[IBIS Ver]   3.2
[File Name]   sprm297.ibs
[File Rev]   1.0
[Date]   November 3, 2003
[Source]   File originated at Texas Instruments
[Copyright]   (c) 2003, Texas Instruments Inc.
[Component]   f2812ghh
[Manufacturer] Texas Instruments
[Package]
| Variable   Typ   Min   Max
R_pkg   0.08821   0.00445   0.1444
L_pkg   2.312e-09   3.373e-10   3.933e-09
C_pkg   2.855e-13   1.279e-13   4.259e-13
[Pin] signal_name   model_name   R_pin   L_pin   C_pin
B2   VDDAIO   NC   0.09209  2.36e-09   2.324e-13
C2   ADCINB0   ioh125   0.08702  2.145e-09  2.491e-13
C3   ADCINB1   ioh125   0.08455  2.129e-09  2.412e-13
B1   ADCINB2   ioh125   0.1237   3.291e-09  3.802e-13
C1   ADCINB3   ioh125   0.103   2.673e-09  3.339e-13
D3   ADCINB4   ioh125   0.07884  2.005e-09  2.389e-13
D2   ADCINB5   ioh125   0.07849  1.946e-09  2.548e-13
D1   ADCINB6   ioh125   0.09972  2.597e-09  2.918e-13
F5   ADCINB7   ioh125   0.1392   3.811e-09  4.225e-13
E4   ADCREFM   ioh125   0.1002   2.62e-09   3.512e-13
E2   ADCREFP   ioh125   0.07253  1.807e-09  2.304e-13
E3   AVSSREFBG   ioh125   0.07152  1.838e-09  2.399e-13
E1   AVDDREFBG   ioh125   0.09207  2.431e-09  2.756e-13
F4   VDDA1   NC   0.09478  2.501e-09  3.059e-13
F3   VSSA1   NC   0.06871  1.775e-09  2.4e-13
F2   ADCRESEXT   ioh125   0.06839  1.711e-09  2.218e-13
F1   XMPNMC   idg095_pe1005   0.09079  2.383e-09  2.69e-13
G5   XA(0)   oui835   0.1124   3.004e-09  3.787e-13
G4   VSS   NC   0.09241  2.449e-09  3.276e-13
G2   MDRA   idg095_ouo435_ps1005  0.06703  1.677e-09  2.109e-13
G3   XD(0)   idg095_oui835_ps1005  0.06663  1.72e-09   2.244e-13
G1   MDXA   idg095_ouo435   0.08649  2.3e-09   3.064e-13
H1   VDD   NC   0.08687  2.308e-09  3.051e-13
H3   XD(1)   idg095_oui835_ps1005  0.0675   1.739e-09  2.278e-13
H2   MCLKRA   idg095_ouo435_ps1005  0.06857  1.71e-09   2.172e-13
H4   MFSXA   idg095_ouo435_ps1005  0.0958   2.514e-09  3.319e-13
H5   XD(2)   idg095_oui835_ps1005  0.1148   3.076e-09  3.819e-13
J1   MCLKXA   idg095_ouo435_ps1005  0.09444  2.462e-09  2.835e-13
J2   MFSRA   idg095_ouo435_ps1005  0.07272  1.804e-09  2.338e-13
J3   XD(3)   idg095_oui835_ps1005  0.07371  1.889e-09  2.436e-13
J4   VDDIO   NC   0.09822  2.576e-09  3.054e-13
K1   VSS   NC   0.09654  2.518e-09  2.844e-13
K3   XD(4)   idg095_oui835_ps1005  0.07688  1.955e-09  2.515e-13
K2   SPICLKA   idg095_ouo435   0.07656  1.898e-09  2.333e-13
K4   SPISTEA   idg095_ouo435   0.1045   2.711e-09  3.594e-13
J5   XD(5)   idg095_oui835_ps1005  0.1444   3.933e-09  4.259e-13
L1   VDD   NC   0.1023   2.666e-09  2.93e-13
L2   VSS   NC   0.08196  2.025e-09  2.536e-13
L3   XD(6)   idg095_oui835_ps1005  0.08003  2.035e-09  2.292e-13
M1   SPISIMOA   idg095_ouo435   0.1022   2.66e-09   3.169e-13
N1   SPISOMIA   idg095_ouo435   0.1206   3.247e-09  3.719e-13
M3   XRDn   oui835   0.08199  2.072e-09  2.38e-13
M2   XA(1)   oui835   0.08514  2.104e-09  2.563e-13
P1   XZCS0AND1n   oui835   0.1272   3.432e-09  3.17e-13
N2   PWM7   sw0145_ouo435_ups285  0.09249  2.375e-09  2.344e-13
P2   PWM8   sw0145_ouo435_ups285  0.1091   2.835e-09  3.24e-13
N3   PWM9   sw0145_ouo435_ups285  0.0847   2.1e-09   2.977e-13
P3   PWM10   sw0145_ouo435_ups285  0.1058   2.786e-09  3.224e-13
L4   PWM11   sw0145_ouo435_ups285  0.1017   2.696e-09  3.056e-13
M4   PWM12   sw0145_ouo435_ups285  0.07819  1.991e-09  2.576e-13
N4   XRNW   oui835   0.07522  1.886e-09  2.531e-13
P4   VSS   NC   0.09848  2.623e-09  3.028e-13
K5   T3PWM_T3CMP   sw0145_ouo435_ups285  0.1128   3.022e-09  3.435e-13
L5   XD(7)   idg095_oui835_ps1005  0.09136  2.382e-09  3.006e-13
N5   T4PWM_T4CMP   sw0145_ouo435_ups285  0.06842  1.716e-09  2.385e-13
P5   VDD   NC   0.09175  2.499e-09  2.855e-13
M5   CAP4_QEP3   sw0145_ouo435_ups285  0.05893  1.5e-09   2.17e-13
K6   VSS   NC   0.1035   2.805e-09  3.409e-13
M6   CAP5_QEP4   sw0145_ouo435_ups285  0.06207  1.604e-09  2.311e-13
P6   CAP6_QEPI2   sw0145_ouo435_ups285  0.09133  2.468e-09  2.967e-13
N6   C4TRIPn   sw0145_ouo435_ups285  0.06341  1.612e-09  2.156e-13
L6   C5TRIPn   sw0145_ouo435_ups285  0.08399  2.26e-09   3.049e-13
K7   C6TRIPn   sw0145_ouo435_ups285  0.1038   2.828e-09  3.985e-13
L7   VDDIO   NC   0.08372  2.239e-09  3.16e-13
P7   XD(8)   idg095_oui835_ps1005  0.0865   2.353e-09  2.75e-13
N7   TEST2   iog195   0.06169  1.56e-09   2.049e-13
M7   TEST1   iog195   0.06268  1.695e-09  2.38e-13
M8   XD(9)   idg095_oui835_ps1005  0.06259  1.694e-09  2.398e-13
N8   VDD3VFL   NC   0.0611   1.546e-09  2.12e-13
P8   VSS   NC   0.08825  2.433e-09  2.701e-13
L8   TDIRB   sw0145_ouo435_ups285  0.08293  2.235e-09  3.129e-13
K8   TCLKINB   sw0145_ouo435_ups285  0.102   2.793e-09  3.815e-13
L9   XD(10)   idg095_oui835_ps1005  0.0859   2.316e-09  3.071e-13
N9   XD(11)   idg095_oui835_ps1005  0.06134  1.562e-09  2.256e-13
P9   VDD   NC   0.08678  2.402e-09  2.814e-13
M9   X2   NC   0.05751  1.488e-09  2.185e-13
K9   X1/XCLKIN   NC   0.1051   2.874e-09  3.416e-13
M10   VSS   NC   0.06466  1.77e-09   2.525e-13
P10   T3CTRIP_PDPINTBn idg095_ouo435_ps1005  0.09255  2.499e-09  2.906e-13
N10   XA(2)   oui835   0.06746  1.702e-09  2.398e-13
L10   VDDIO   NC   0.09217  2.446e-09  3.236e-13
K10   XHOLDAn   oui835   0.1143   3.12e-09   3.69e-13
P11   T4CTRIPn/EVBSOCn idg095_ouo435_ps1005  0.09684  2.574e-09  2.997e-13
N11   XWEn   oui835   0.07403  1.857e-09  2.454e-13
M11   XA(3)   oui835   0.07441  1.903e-09  2.389e-13
L11   VSS   NC   0.104   2.76e-09   3.07e-13
P12   VDD   NC   0.103   2.706e-09  3.157e-13
N12   CANTXA   idg095_ouo435_ps1005  0.08258  2.052e-09  2.669e-13
P13   XZCS2n   oui835   0.1083   2.856e-09  2.829e-13
N13   CANRXA   idg095_ouo435_ps1005  0.09197  2.37e-09   2.499e-13
P14   SCITXDB   idg095_ouo435   0.1255   3.388e-09  3.392e-13
M13   SCIRXDB   idg095_ouo435   0.08237  2.039e-09  2.548e-13
M12   PWM1   idg095_ouo435_ps1005  0.08225  2.075e-09  2.456e-13
N14   VDDIO   NC   0.1201   3.231e-09  3.81e-13
M14   PWM2   idg095_ouo435_ps1005  0.09891  2.59e-09   3.294e-13
L12   PWM3   idg095_ouo435_ps1005  0.07898  2.006e-09  2.447e-13
L13   PWM4   idg095_ouo435_ps1005  0.07487  1.867e-09  2.444e-13
L14   XD(12)   idg095_oui835_ps1005  0.09893  2.587e-09  2.886e-13
J10   XD(13)   idg095_oui835_ps1005  0.1386   3.798e-09  4.176e-13
K11   PWM5   idg095_ouo435_ps1005  0.09954  2.607e-09  3.482e-13
K13   VSS   NC   0.0709   1.771e-09  2.325e-13
K12   VDD   NC   0.07034  1.811e-09  2.401e-13
K14   PWM6   idg095_ouo435_ps1005  0.09406  2.475e-09  2.775e-13
J11   T1PWM_T1CMP   idg095_ouo435_ps1005  0.09311  2.447e-09  3.027e-13
J12   XA(4)   oui835   0.0707   1.815e-09  2.418e-13
J13   T2PWM_T2CMP   idg095_ouo435_ps1005  0.06707  1.681e-09  2.219e-13
J14   VSS   NC   0.09108  2.388e-09  2.791e-13
H10   CAP1_QEP1   idg095_ouo435_ps1005  0.1139   3.036e-09  3.844e-13
H11   CAP2_QEP2   idg095_ouo435_ps1005  0.09328  2.466e-09  3.308e-13
H13   XA(5)   oui835   0.06503  1.629e-09  2.144e-13
H12   CAP3_QEPI1   idg095_ouo435_ps1005  0.06577  1.702e-09  2.25e-13
H14   T1CTRIP_PDPINTAn idg095_ouo435_ps1005  0.08639  2.297e-09  3.03e-13
G14   XA(6)   oui835   0.0873   2.319e-09  3.041e-13
G12   VDD   NC   0.06918  1.777e-09  2.274e-13
G13   VSS   NC   0.06778  1.692e-09  2.146e-13
G11   VDDIO   NC   0.09314  2.459e-09  3.346e-13
G10   T2CTRIPn/EVASOCn idg095_ouo435_ps1005  0.1138   3.052e-09  3.802e-13
F14   TDIRA   idg095_ouo435_ps1005  0.09404  2.462e-09  2.798e-13
F13   TCLKINA   idg095_ouo435_ps1005  0.06786  1.696e-09  2.218e-13
F12   XA(7)   oui835   0.07232  1.856e-09  2.474e-13
F11   XCLKOUT   oui835   0.09426  2.507e-09  3.058e-13
E14   VSS   NC   0.09525  2.497e-09  2.91e-13
E12   XA(8)   oui835   0.07626  1.938e-09  2.582e-13
E13   C1TRIPn   idg095_ouo435_ps1005  0.07579  1.878e-09  2.366e-13
E11   C2TRIPn   idg095_ouo435_ps1005  0.1028   2.672e-09  3.561e-13
F10   C3TRIPn   idg095_ouo435_ps1005  0.1414   3.864e-09  4.252e-13
D14   XA(9)   oui835   0.1035   2.69e-09   2.981e-13
D13   TMS   idg095_ps1005   0.07795  1.936e-09  2.479e-13
D12   TDO   oui835   0.08151  2.062e-09  2.503e-13
C14   VDD   NC   0.1046   2.725e-09  3.442e-13
B14   VSS   NC   0.1242   3.313e-09  3.855e-13
C12   XA(10)   oui835   0.08905  2.226e-09  2.563e-13
C13   TDI   idg095_ps1005   0.0903   2.216e-09  2.631e-13
A14   XA(11)   oui835   0.1281   3.455e-09  3.132e-13
B13   XZCS6AND7n   oui835   0.09387  2.397e-09  2.377e-13
A13   TESTSEL   idg095_pe1005   0.1042   2.726e-09  3.249e-13
B12   TRSTn   idg095_pe1005   0.00445  3.373e-10  1.279e-13
A12   TCK   idg095_ps1005   0.1012   2.679e-09  3.184e-13
D11   EMU0   idg095_oui835_ps1005  0.09979  2.649e-09  3.147e-13
C11   XA(12)   oui835   0.07303  1.881e-09  2.526e-13
B11   XD(14)   idg095_oui835_ps1005  0.07161  1.807e-09  2.388e-13
A11   XF_XPLLDIS   idg095_oui835_ps1005  0.09603  2.567e-09  2.922e-13
E10   XA(13)   oui835   0.1156   3.087e-09  3.455e-13
D10   VSS   NC   0.09186  2.405e-09  2.985e-13
B10   VDD   NC   0.06885  1.731e-09  2.29e-13
A10   XA(14)   oui835   0.09485  2.561e-09  2.856e-13
C10   VSS   NC   0.063988 1.613e-09  2.243e-13
E9   VDDIO   NC   0.1082   2.906e-09  3.452e-13
C9   EMU1   idg095_oui835_ps1005  0.06274  1.614e-09  2.346e-13
A9   XD(15)   idg095_oui835_ps1005  0.09338  2.506e-09  3.182e-13
B9   XA(15)   oui835   0.06408  1.62e-09   2.367e-13
D9   XINT1_XBIOn   idg095_ouo435   0.08668  2.311e-09  3.397e-13
E8   XNMI_XINT13   idg095_ouo435_ps1005  0.1043   2.833e-09  3.974e-13
D8   XINT2_ADCSOC   idg095_ouo435   0.08381  2.248e-09  3.111e-13
A8   XA(16)   oui835   0.08698  2.367e-09  2.747e-13
B8   VSS   NC   0.06146  1.548e-09  2.203e-13
C8   VDD   NC   0.0627   1.691e-09  2.545e-13
C7   SCITXDA   idg095_ouo435_ps1005  0.06257  1.689e-09  2.491e-13
B7   XA(17)   oui835   0.06157  1.552e-09  2.151e-13
A7   SCIRXDA   idg095_ouo435_ps1005  0.08827  2.43e-09   2.835e-13
D7   XA(18)   oui835   0.08506  2.269e-09  3.34e-13
E7   XHOLDn   idg095_ps1005   0.1043   2.826e-09  3.994e-13
D6   XRSn   idg095_oum425_ps1005  0.08576  2.305e-09  3.177e-13
B6   XREADY   idg095_ps1005   0.0641   1.621e-09  2.324e-13
A6   VDD1   NC   0.09005  2.472e-09  2.845e-13
C6   VSS1   NC   0.06117  1.569e-09  2.29e-13
E6   ADCBGREFIN   ioh125   0.1067   2.898e-09  3.505e-13
C5   VSSA2   NC   0.06463  1.768e-09  2.521e-13
A5   VDDA2   NC   0.09355  2.521e-09  2.935e-13
B5   ADCINA7   ioh125   0.06979  1.749e-09  2.589e-13
D5   ADCINA6   ioh125   0.09531  2.493e-09  3.268e-13
E5   ADCINA5   ioh125   0.115   3.131e-09  3.515e-13
A4   ADCINA4   ioh125   0.101   2.662e-09  3.031e-13
B4   ADCINA3   ioh125   0.07696  1.923e-09  2.515e-13
C4   ADCINA2   ioh125   0.0785   1.993e-09  2.483e-13
D4   ADCINA1   ioh125   0.1037   2.755e-09  3.086e-13
A3   ADCINA0   ioh125   0.1053   2.763e-09  3.109e-13
B3   ADCLO   ioh125   0.08665  2.149e-09  2.561e-13
A2   VSSAIO   NC   0.1087   2.841e-09  2.701e-13
| End of package information
| Component idg095
[Component]   idg095
[Manufacturer]   Texas Instruments
[Package]
|   typ   min   max
R_pkg   0   0   0
L_pkg   0   0   0
C_pkg   0   0   0
[Pin]   signal_name   model_name   R_pin   L_pin   C_pin
   1   A   idg095   0   0   0
| Component idg095_oui835_ps1005
[Component]   idg095_oui835_ps1005
[Manufacturer]   Texas Instruments
[Package]
|   typ   min   max
R_pkg   0   0   0
L_pkg   0   0   0
C_pkg   0   0   0
[Pin]   signal_name   model_name   R_pin   L_pin   C_pin
   1   Y  idg095_oui835_ps1005   0   0   0
| Component idg095_oum425_ps1005
[Component]   idg095_oum425_ps1005
[Manufacturer]   Texas Instruments
[Package]
|   typ   min   max
R_pkg   0   0   0
L_pkg   0   0   0
C_pkg   0   0   0
[Pin]   signal_name   model_name   R_pin   L_pin   C_pin
   1   Y  idg095_oum425_ps1005   0   0   0
| Component idg095_ouo435_ps1005
[Component]   idg095_ouo435_ps1005
[Manufacturer]   Texas Instruments
[Package]
|   typ   min   max
R_pkg   0   0   0
L_pkg   0   0   0
C_pkg   0   0   0
[Pin]   signal_name   model_name   R_pin   L_pin   C_pin
   1   Y  idg095_ouo435_ps1005   0   0   0
| Component idg095_pe1005
[Component]   idg095_pe1005
[Manufacturer]   Texas Instruments
[Package]
|   typ   min   max
R_pkg   0   0   0
L_pkg   0   0   0
C_pkg   0   0   0
[Pin]   signal_name   model_name   R_pin   L_pin   C_pin
   1   A   idg095_pe1005   0   0   0
| Component idg095_ps1005
[Component]   idg095_ps1005
[Manufacturer]   Texas Instruments
[Package]
|   typ   min   max
R_pkg   0   0   0
L_pkg   0   0   0
C_pkg   0   0   0
[Pin]   signal_name   model_name   R_pin   L_pin   C_pin
   1   A   idg095_ps1005   0   0   0
| Component iog195
[Component]   iog195
[Manufacturer]   Texas Instruments
[Package]
|   typ   min   max
R_pkg   0   0   0
L_pkg   0   0   0
C_pkg   0   0   0
[Pin]   signal_name   model_name   R_pin   L_pin   C_pin
   1   Y   iog195   0   0   0
| Component ioh125
[Component]   ioh125
[Manufacturer]   Texas Instruments
[Package]
|   typ   min   max
R_pkg   0   0   0
L_pkg   0   0   0
C_pkg   0   0   0
[Pin]   signal_name   model_name   R_pin   L_pin   C_pin
   1   Y   ioh125   0   0   0
| Component oui835
[Component]   oui835
[Manufacturer]   Texas Instruments
[Package]
|   typ   min   max
R_pkg   0   0   0
L_pkg   0   0   0
C_pkg   0   0   0
[Pin]   signal_name   model_name   R_pin   L_pin   C_pin
   1   Y   oui835   0   0   0
| Component oum425
[Component]   oum425
[Manufacturer]   Texas Instruments
[Package]
|   typ   min   max
R_pkg   0   0   0
L_pkg   0   0   0
C_pkg   0   0   0
[Pin]   signal_name   model_name   R_pin   L_pin   C_pin
   1   Y   oum425   0   0   0
| Component idg095_ouo435
[Component]   idg095_ouo435
[Manufacturer]   Texas Instruments
[Package]
|   typ   min   max
R_pkg   0   0   0
L_pkg   0   0   0
C_pkg   0   0   0
[Pin]   signal_name   model_name   R_pin   L_pin   C_pin
   1   Y   idg095_ouo435   0   0   0
| Component ouo435
[Component]   ouo435
[Manufacturer]   Texas Instruments
[Package]
|   typ   min   max
R_pkg   0   0   0
L_pkg   0   0   0
C_pkg   0   0   0
[Pin]   signal_name   model_name   R_pin   L_pin   C_pin
   1   Y   ouo435   0   0   0
| Component sw0145_ouo435_ups285
[Component]   sw0145_ouo435_ups285
[Manufacturer]   Texas Instruments
[Package]
|   typ   min   max
R_pkg   0   0   0
L_pkg   0   0   0
C_pkg   0   0   0
[Pin]   signal_name   model_name   R_pin   L_pin   C_pin
   1   Y  sw0145_ouo435_ups285   0   0   0
| Models and submodels in the file (13): idg095 (Input), idg095_oui835_ps1005 (I/O), idg095_oum425_ps1005 (I/O_open_sink), idg095_ouo435_ps1005 (I/O), idg095_pe1005 (Input), idg095_ps1005 (Input), iog195 (Terminator), ioh125 (Terminator), oui835 (3-state), oum425 (I/O_open_sink), idg095_ouo435 (I/O), ouo435 (3-state), sw0145_ouo435_ups285 (I/O)
